(* Logix 5000 DataType export DriveStatus; software revision 24.00 *)

TYPE DriveStatus :
STRUCT
   Drive_Enable : BOOL;   // Drive Enable Input
   Drive_Homed : BOOL;   // Drive Home Input
   Drive_InMotion : BOOL;   // Drive In Motion Input
   Drive_EStop : BOOL;   // Drive E-Stop Input
   rsved_bit00 : BOOL;
   rsved_bit01 : BOOL;
   rsved_bit02 : BOOL;
   rsved_bit03 : BOOL;
   rsved_bit04 : BOOL;
   rsved_bit05 : BOOL;
   rsved_bit06 : BOOL;
   rsved_bit07 : BOOL;
   rsved_bit08 : BOOL;
   Drive_EthAvail : BOOL;   // Drive Ethernet Online
   rsved_bit09 : BOOL;
   rsved_bit10 : BOOL;
   rsved_bit11 : BOOL;
   rsved_bit12 : BOOL;
   rsved_bit13 : BOOL;
   rsved_bit14 : BOOL;
   Drive_BrakeOff : BOOL;   // Brake Output (0 - Enabled; 1- Not Enabled)
   rsved_bit15 : BOOL;
   rsved_bit16 : BOOL;
   rsved_bit17 : BOOL;
   Drive_IdxActive : BOOL;   // Indexer Active
   Drive_IdxPaused : BOOL;   // Indexer Paused
   rsrved_bit20 : BOOL;
   rsrved_bit21 : BOOL;
   rsrved_bit22 : BOOL;
   rsrved_bit23 : BOOL;
   rsrved_bit24 : BOOL;
   Drive_HostControl : BOOL;   // Software In Control - Ignoring Network Commands (example: Tolomatic Motion Interface)
END_STRUCT
END_TYPE
